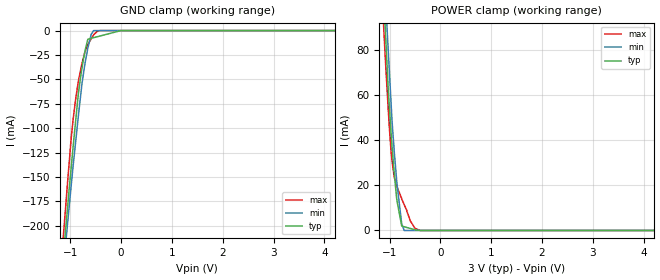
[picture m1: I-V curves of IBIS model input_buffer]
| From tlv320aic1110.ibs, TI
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|   input_buffer Model
[Model]   input_buffer
Model_type   Input
Vinl = 0.9
Vinh = 2.1
|   typ   min   max
|   (nom PVT)   (Fast PVT)   (slow PVT)
|Average
C_comp   1.513e-12   1.510e-12   1.516e-12
| Where nom  PVT is Nominal Process,  3V,  65C
|   Fast PVT is Strong Process,   3.3V,  -40C
|   Slow PVT is Weak Process,   2.7V,  125C
[Model Spec]
|   typ   min   max
Vinl   0.9   0.81   0.99
Vinh   2.1   1.89   2.31
[Voltage Range]   3   2.7   3.3
|Ambient Temperature   25   105   -40
|Junction Temperature
[Temperature Range]   65   125   -40
[Power Clamp Reference]   3   2.7   3.3
[GND Clamp Reference]   0   0   0
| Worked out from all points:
|   POWER clamp passes 1 mA (typ) near -0.61 V on its own axis
[GND Clamp]
|   Voltage   I(typ)   I(min)   I(max)
-3V       -1.504A    -1.434A    -1.593A
-1.149V   -238.2mA   -250.4mA   -218.3mA
-1.066V   -188.6mA   -204.4mA   -163.5mA
-980.4mV  -138.9mA   -157.5mA   -108.7mA
-944.1mV  -118.7mA   -138.3mA   -90.78mA
-846mV    -66.77mA   -89.65mA   -53.35mA
-798mV    -47.7mA    -67.06mA   -40.53mA
-721.2mV  -23.86mA   -36.95mA   -23.45mA
-654mV    -8.788mA   -17.76mA   -14.13mA
-541.5mV  -7.269mA   0A         -4.37mA
-3.6mV    0A         0A         0A
6V        0A         0A         0A
[POWER Clamp]
|   Voltage   I(typ)   I(min)   I(max)
-3V       1.168A     1.122A     1.28A
-1.129V   110.3mA    125.3mA    96.23mA
-1.079V   87.55mA    103.5mA    74.86mA
-1.042V   70.6mA     87.17mA    60.53mA
-967.2mV  42.61mA    55.68mA    34.6mA
-911.1mV  26.48mA    36.38mA    24.34mA
-861mV    14.57mA    22.73mA    20.03mA
-761.7mV  2.197mA    3.308mA    14.22mA
-710.4mV  1.645mA    0A         11.37mA
-584.4mV  856.5uA    0A         3.989mA
-393mV    0A         0A         0A
6V        0A         0A         0A
